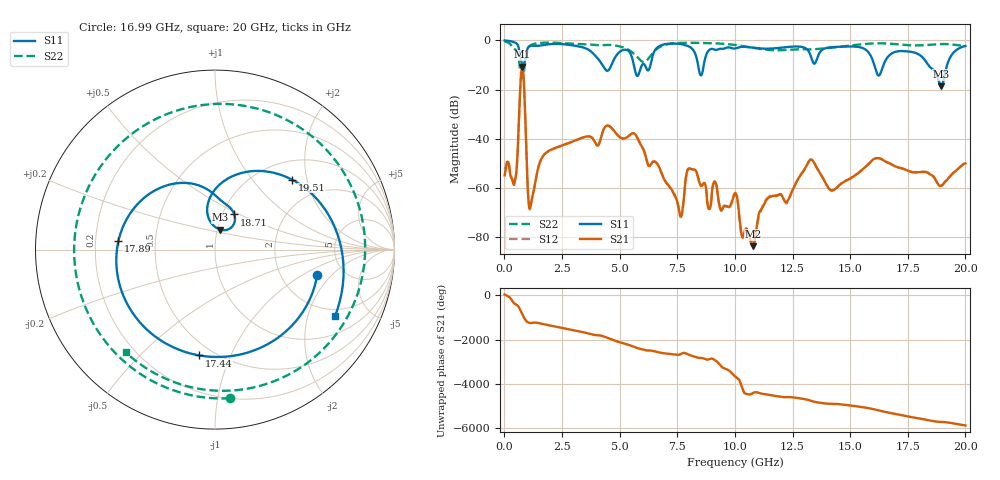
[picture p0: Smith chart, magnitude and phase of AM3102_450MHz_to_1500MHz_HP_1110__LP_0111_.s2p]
!Agilent Technologies,E8364B,MY43040894,A.07.50.67
!Agilent E8364B: A.07.50.67
!Date: Thursday, January 11, 2018 06:43:58
!Correction: S11(Full 2 Port(1,2))
!S21(Full 2 Port(1,2))
!S12(Full 2 Port(1,2))
!S22(Full 2 Port(1,2))
!S2P File: Measurements: S11, S21, S12, S22:
# Hz S  dB  R 50
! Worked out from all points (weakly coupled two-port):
!   1601 points, 10 MHz to 20 GHz, reference 50 ohm
!   highest |S21| = -10.71 dB at 772.1 MHz (marker M1); lowest = -83.6 dB at 10.78 GHz (marker M2)
!   lowest |S11| = -18.7 dB at 18.95 GHz (marker M3), VSWR 1.26, Z = 51.7 + j11.7 ohm
!   |S11| at or under -10 dB: 4.252 GHz to 4.648 GHz (396.4 MHz wide, 8.91 % of centre); 16.05 GHz to 16.45 GHz (401.9 MHz wide, 2.47 % of centre); 18.39 GHz to 19.21 GHz (822.7 MHz wide, 4.38 % of centre)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
!   |S22| runs from -15.2 to -0.4 dB; largest |S21 - S12| = 0.00093
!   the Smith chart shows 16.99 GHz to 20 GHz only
!   S11 on the Smith chart (normalised r, x): 16.99 GHz: 3.20, -1.37; 17.44 GHz: 0.42, -0.77; 17.89 GHz: 0.30, +0.04; 18.71 GHz: 1.14, +0.47; 19.51 GHz: 1.39, +1.63; 20 GHz: 1.68, -3.00
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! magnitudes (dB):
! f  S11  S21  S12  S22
! 10 MHz  -0.1  -54.9  -52.5  -0.4
! 459.8 MHz  -0.9  -57.0  -56.8  -3.7
! 772.1 MHz  -10.1  -10.7  -10.7  -14.8
! 1.122 GHz  -2.3  -68.1  -68.4  -2.2
! 1.709 GHz  -1.9  -46.7  -46.6  -1.0
! 3.346 GHz  -2.8  -39.7  -39.7  -1.6
! 5.77 GHz  -14.5  -39.6  -39.6  -6.8
! 6.682 GHz  -2.6  -50.9  -50.9  -3.1
! 7.644 GHz  -1.5  -71.4  -71.9  -1.1
! 8.043 GHz  -2.7  -52.1  -52.0  -1.0
! 10.01 GHz  -3.4  -62.2  -62.0  -1.9
! 10.78 GHz  -3.0  -83.6  -81.9  -3.0
! 13.34 GHz  -7.8  -48.6  -48.5  -3.7
! 14.24 GHz  -2.8  -61.0  -61.0  -3.0
! 16.68 GHz  -6.4  -49.9  -49.8  -1.4
! 16.99 GHz  -4.6  -51.3  -51.3  -1.6
! 17.44 GHz  -4.5  -52.7  -52.6  -2.0
! 17.89 GHz  -5.3  -53.7  -53.6  -2.1
! 18.71 GHz  -13.0  -56.8  -56.9  -1.7
! 18.95 GHz  -18.7  -59.1  -59.1  -1.6
! 19.51 GHz  -4.7  -53.6  -53.5  -1.8
! 20 GHz  -2.3  -50.0  -49.9  -2.4
